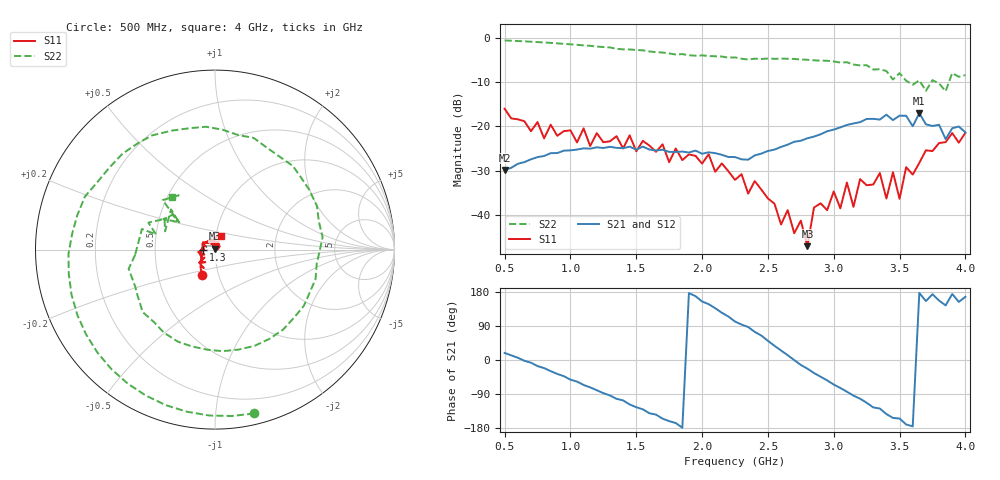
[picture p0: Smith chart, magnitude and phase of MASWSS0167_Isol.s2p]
!Part No	MASWSS0167
!Fixture No	1000013396 REV B
! 2/8/2007  1:06:50 PM	Sample Board de-embdedding pS of delay  RFC 107.1	RF1 109.6
!EA:	CMS
!File Comment	AQTN 1888
!MASWSS0167_3V_4T_CMS.txt	MASWSS0167_4T_ testtitle_A
!Power Level	-5
!Test#	1	1	 Comments
!Fixture Loss is only removed from dB data
!measured state	RF to RF 1 IL
! Created Fri Feb 09 13:31:33 2007
!PORT 1= RFC  PORT2 = RF1
# hz S db R 50
! 2 Port Network Data from SP1.SP block
! freq  dbS11  angS11  dbS21  angS21  dbS12  angS12  dbS22  angS22
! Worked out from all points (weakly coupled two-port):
!   71 points, 500 MHz to 4 GHz, reference 50 ohm
!   highest |S21| = -17.01 dB at 3.65 GHz (marker M1); lowest = -29.9 dB at 500 MHz (marker M2)
!   lowest |S11| = -47.1 dB at 2.8 GHz (marker M3), VSWR 1.01, Z = 50 + j0.438 ohm
!   |S11| at or under -10 dB: start of sweep to end of sweep
!   |S22| runs from -12.0 to -0.5 dB; largest |S21 - S12| = 0.00028
!   S11 on the Smith chart (normalised r, x): 500 MHz: 0.83, -0.24; 1.3 GHz: 0.87, -0.01; 4 GHz: 1.05, +0.17
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5e8  -16.00 -117.4  -29.86 18.6  -29.87 18.6  -0.55 -76.5
8e8  -22.71 -142.9  -26.71 -21.4  -26.73 -21.3  -1.00 -123.0
1.1e9  -20.44 -171.7  -24.96 -65.9  -24.96 -65.9  -1.66 -170.5
1.3e9  -23.38 -177.3  -24.62 -93.6  -24.62 -93.7  -2.13 157.8
1.7e9  -24.06 108.0  -25.29 -154.8  -25.30 -154.9  -3.27 94.1
2.25e9  -32.10 47.7  -26.94 101.5  -26.94 101.6  -4.38 6.7
2.7e9  -44.18 -97.1  -23.48 -0.3  -23.48 -0.3  -4.73 -67.7
2.75e9  -41.33 110.1  -23.25 -13.0  -23.25 -13.0  -4.85 -76.8
2.8e9  -47.11 95.8  -22.68 -23.0  -22.68 -23.0  -4.92 -85.6
2.85e9  -38.38 132.6  -22.31 -34.4  -22.31 -34.3  -5.04 -94.2
3e9  -34.72 84.8  -20.73 -64.8  -20.72 -64.7  -5.30 -121.7
3.05e9  -38.55 105.8  -20.22 -73.8  -20.22 -73.7  -5.55 -129.8
3.1e9  -32.70 93.4  -19.68 -83.7  -19.66 -83.7  -5.48 -139.2
3.15e9  -38.22 85.7  -19.34 -94.0  -19.33 -94.0  -6.00 -149.5
3.2e9  -31.94 111.1  -19.04 -102.1  -19.02 -102.2  -6.20 -155.2
3.35e9  -30.56 68.9  -18.45 -128.1  -18.44 -128.1  -7.05 -177.0
3.4e9  -36.34 100.5  -17.35 -142.6  -17.34 -142.7  -7.47 164.2
3.45e9  -30.36 90.0  -18.58 -152.8  -18.57 -152.9  -9.39 165.6
3.5e9  -36.41 100.6  -17.57 -154.5  -17.57 -154.6  -7.95 158.0
3.55e9  -29.23 111.2  -17.60 -170.1  -17.60 -170.2  -9.66 148.7
3.65e9  -28.26 124.4  -17.01 177.0  -17.00 176.9  -9.58 137.6
4e9  -21.46 67.3  -21.35 166.7  -21.34 166.6  -8.39 129.5
